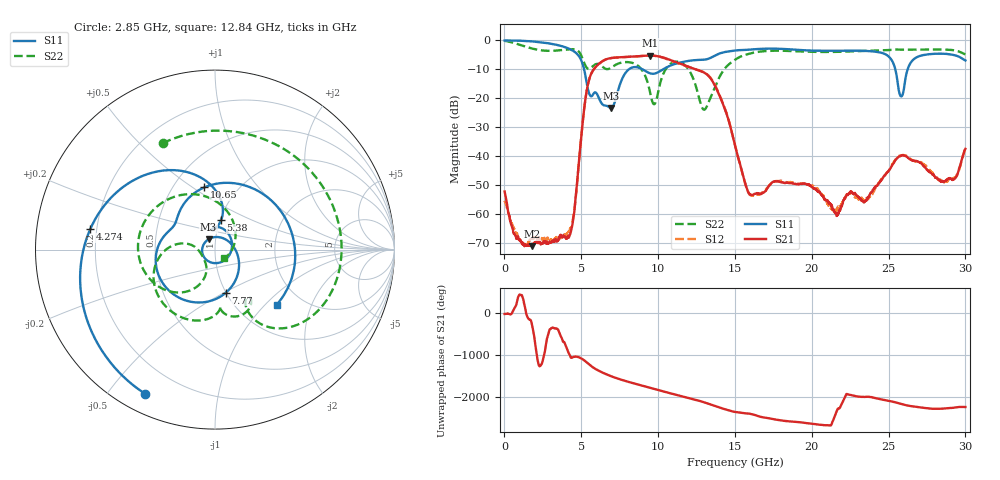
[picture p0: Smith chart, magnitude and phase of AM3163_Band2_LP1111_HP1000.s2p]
!Agilent Technologies,E8364B,MY43040894,A.07.50.67
!Agilent E8364B: A.07.50.67
!Date: Thursday, August 20, 2020 12:09:57
!Correction: S11(Full 2 Port(1,2))
!S21(Full 2 Port(1,2))
!S12(Full 2 Port(1,2))
!S22(Full 2 Port(1,2))
!S2P File: Measurements: S11, S21, S12, S22:
# Hz S  dB  R 50
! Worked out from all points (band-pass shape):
!   3201 points, 10 MHz to 30 GHz, reference 50 ohm
!   highest |S21| = -5.23 dB at 9.457 GHz (marker M1); lowest = -71.2 dB at 1.772 GHz (marker M2)
!   |S21| within 3 dB of the highest: 6.119 GHz to 11.53 GHz (5.408 GHz wide, 61.3 % of centre)
!   lowest |S11| = -23.4 dB at 6.926 GHz (marker M3), VSWR 1.15, Z = 46.3 + j5.36 ohm
!   |S11| at or under -10 dB: 5.184 GHz to 8.096 GHz (2.911 GHz wide, 43.8 % of centre); 8.983 GHz to 10.33 GHz (1.345 GHz wide, 13.9 % of centre); 25.44 GHz to 26.24 GHz (801.9 MHz wide, 3.1 % of centre)
!   |S22| runs from -24.0 to -0.1 dB; largest |S21 - S12| = 0.013
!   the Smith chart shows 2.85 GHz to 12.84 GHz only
!   S11 on the Smith chart (normalised r, x): 2.85 GHz: 0.08, -0.62; 4.274 GHz: 0.17, +0.08; 5.38 GHz: 1.01, +0.34; 7.77 GHz: 1.00, -0.51; 10.65 GHz: 0.71, +0.56; 12.84 GHz: 1.50, -1.17
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1e7  -0.02 -2.8  -52.24 -21.0  -55.45 69.4  -0.15 -6.9
8.440969e8  -0.08 -33.3  -68.31 -45.4  -67.45 -130.2  -1.25 -80.8
1.771912e9  -0.33 -70.6  -71.18 116.2  -68.92 72.6  -2.77 -160.0
2.849678e9  -0.99 -116.0  -70.24 -144.9  -68.51 -5.3  -3.61 116.2
4.274203e9  -3.04 170.7  -67.03 54.2  -65.04 105.8  -3.05 10.9
5.014581e9  -7.09 106.8  -32.44 -3.6  -32.42 -3.9  -5.42 -54.3
5.380084e9  -15.53 78.3  -16.59 -107.2  -16.63 -107.4  -9.60 -59.1
6.092347e9  -19.27 36.5  -8.36 71.3  -8.42 71.1  -8.13 -70.8
6.926444e9  -23.37 121.7  -6.11 -65.4  -6.14 -65.6  -9.49 -85.5
7.769912e9  -12.13 -75.7  -5.74 -169.8  -5.79 -169.6  -7.54 -114.4
9.45685e9  -11.36 154.8  -5.23 17.2  -5.22 17.1  -17.46 168.9
1.000979e10  -10.99 136.6  -5.50 -38.6  -5.52 -39.1  -17.71 -111.7
1.064708e10  -9.07 99.7  -6.46 -101.3  -6.63 -101.8  -8.87 -141.9
1.28401e10  -6.72 -41.9  -10.74 48.2  -10.71 49.6  -22.97 -42.8
1.5005e10  -3.51 -132.4  -36.42 160.0  -36.34 159.7  -6.70 -112.2
1.599842e10  -3.17 -173.9  -53.39 115.8  -53.49 116.8  -4.51 -172.1
1.787279e10  -2.89 98.2  -48.90 -37.0  -48.62 -38.5  -3.57 92.3
2.000958e10  -3.52 -9.9  -50.68 -122.0  -50.29 -120.8  -3.94 -9.3
2.230569e10  -3.56 -99.8  -53.25 -134.4  -52.92 -132.6  -3.86 -93.5
2.500479e10  -5.56 158.0  -45.17 64.6  -45.09 66.6  -3.35 -167.6
2.582014e10  -19.37 170.9  -39.93 -8.9  -39.79 -6.9  -3.20 170.4
3e10  -6.93 54.9  -37.51 -83.3  -37.37 -87.5  -4.84 55.5
